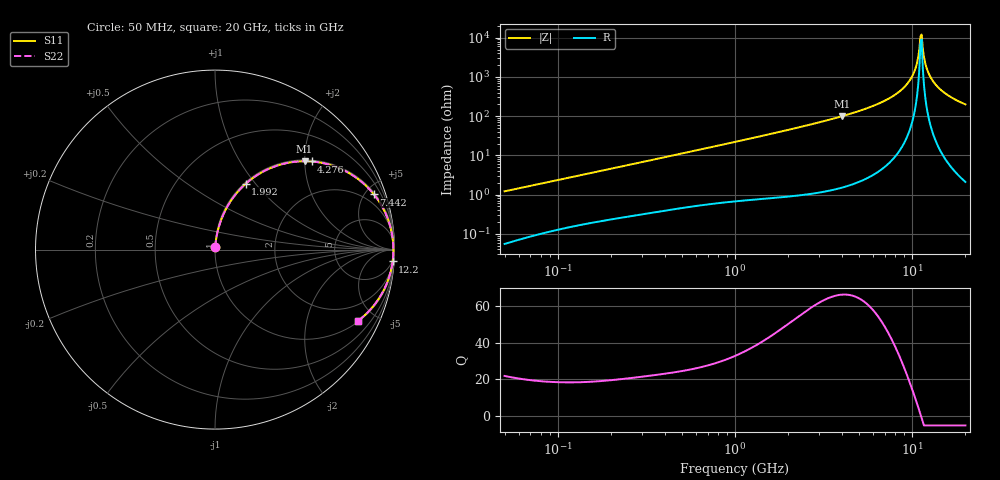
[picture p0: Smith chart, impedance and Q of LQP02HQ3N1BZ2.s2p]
!Murata Part Number: LQP02HQ3N1BZ2
!These Parameters are Measured in Series Mode Connection
!  o--[Z]--o
!Port1  Port2
!  o-------o
!Freq. Start=50[MHz] Stop=20[GHz], 401[Steps]
# Hz S RI R 50
!Freq.(Hz) S11(Real) S11(Imag) S21(Real) S21(Imag) S12(Real) S12(Imag) S22(Real) S22(Imag)
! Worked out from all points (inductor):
!   401 points, 50 MHz to 20 GHz, reference 50 ohm
!   read as one part in series: L = 3.82 nH near 51.52 MHz
!   highest Q = 66.1 at 4.027 GHz (marker M1), where L = 3.95 nH
!   self-resonance near 11.15 GHz
!   S11 on the Smith chart (normalised r, x): 50 MHz: 1.00, +0.02; 1.992 GHz: 1.02, +0.89; 4.276 GHz: 1.03, +2.16; 7.442 GHz: 1.13, +5.72; 12.2 GHz: 4, -29; 20 GHz: 1.04, -3.99
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5e7  0.0007 0.0121  0.9993 -0.0121  0.9993 -0.0121  0.0007 0.0121
1.364002e8  0.00271 0.0316  0.9973 -0.0316  0.9973 -0.0316  0.00271 0.0316
3.721004e8  0.0105 0.0824  0.9895 -0.0824  0.9895 -0.0824  0.0105 0.0824
1e9  0.0521 0.2075  0.9479 -0.2075  0.9479 -0.2075  0.0521 0.2075
1.99176e9  0.1707 0.3664  0.8293 -0.3664  0.8293 -0.3664  0.1707 0.3664
2.728004e9  0.2856 0.4434  0.7144 -0.4434  0.7144 -0.4434  0.2856 0.4434
4.026975e9  0.4992 0.4925  0.5008 -0.4925  0.5008 -0.4925  0.4992 0.4925
4.275624e9  0.5379 0.4911  0.4621 -0.4911  0.4621 -0.4911  0.5379 0.4911
5.856089e9  0.7472 0.4262  0.2528 -0.4262  0.2528 -0.4262  0.7472 0.4262
7.442007e9  0.8856 0.3072  0.1144 -0.3072  0.1144 -0.3072  0.8856 0.3072
8.774992e9  0.953 0.1952  0.047 -0.1952  0.047 -0.1952  0.953 0.1952
9.892087e9  0.9826 0.1033  0.0174 -0.1033  0.0174 -0.1033  0.9826 0.1033
1.050288e10  0.9906 0.0553  0.00944 -0.0553  0.00944 -0.0553  0.9906 0.0553
1.098561e10  0.9934 0.0189  0.00658 -0.0189  0.00658 -0.0189  0.9934 0.0189
1.115139e10  0.9938 0.00675  0.00623 -0.00675  0.00623 -0.00675  0.9938 0.00675
1.149051e10  0.9936 -0.0176  0.00641 0.0176  0.00641 0.0176  0.9936 -0.0176
1.183995e10  0.9922 -0.0419  0.0078 0.0419  0.0078 0.0419  0.9922 -0.0419
1.220001e10  0.9896 -0.0662  0.0104 0.0662  0.0104 0.0662  0.9896 -0.0662
1.314879e10  0.978 -0.1258  0.022 0.1258  0.022 0.1258  0.978 -0.1258
1.460232e10  0.9499 -0.2056  0.0501 0.2056  0.0501 0.2056  0.9499 -0.2056
1.696185e10  0.888 -0.3076  0.112 0.3076  0.112 0.3076  0.888 -0.3076
2e10  0.7968 -0.3971  0.2032 0.3971  0.2032 0.3971  0.7968 -0.3971
